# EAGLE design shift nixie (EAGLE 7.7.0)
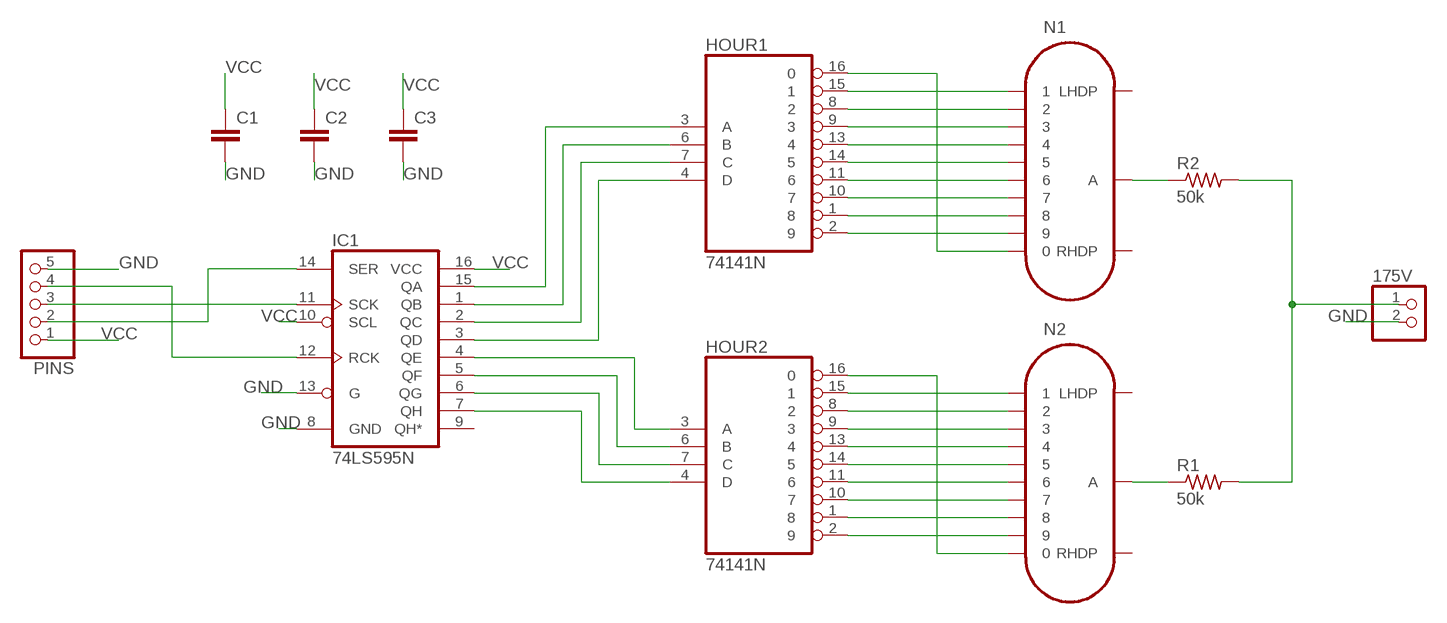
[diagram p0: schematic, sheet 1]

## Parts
175V  PINHD-1X2  [1X02]
C1  CAPPTH  [CAP-PTH-SMALL]
C2  CAPPTH  [CAP-PTH-SMALL]
C3  CAPPTH  [CAP-PTH-SMALL]
HOUR1  74141N  [DIL16]
HOUR2  74141N  [DIL16]
IC1  74LS595N  [DIL16]
N1  IN-14  [IN-14]
N2  IN-14  [IN-14]
PINS  PINHD-1X5  [1X05]
R1  50k  R-US_0204/7  [0204/7]
R2  50k  R-US_0204/7  [0204/7]

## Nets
GND: 175V.2 C1.2 C2.2 C3.2 IC1.8(GND) IC1.13(G) PINS.5
N$1: IC1.11(SCK) PINS.3
N$2: IC1.14(SER) PINS.2
N$3: IC1.12(RCK) PINS.4
N$4: HOUR1.3(A) IC1.15(QA)
N$5: HOUR1.6(B) IC1.1(QB)
N$6: HOUR1.7(C) IC1.2(QC)
N$7: HOUR1.4(D) IC1.3(QD)
N$8: HOUR2.3(A) IC1.4(QE)
N$9: HOUR2.6(B) IC1.5(QF)
N$10: HOUR2.7(C) IC1.6(QG)
N$11: HOUR2.4(D) IC1.7(QH)
N$12: HOUR2.15 N2.1
N$13: HOUR2.8 N2.2
N$14: HOUR2.9 N2.3
N$15: HOUR2.13 N2.4
N$16: HOUR2.14 N2.5
N$17: HOUR2.11 N2.6
N$18: HOUR2.10 N2.7
N$19: HOUR2.1 N2.8
N$20: HOUR2.2 N2.9
N$21: HOUR2.16 N2.0
N$22: HOUR1.15 N1.1
N$23: HOUR1.8 N1.2
N$24: HOUR1.9 N1.3
N$25: HOUR1.13 N1.4
N$26: HOUR1.14 N1.5
N$27: HOUR1.11 N1.6
N$28: HOUR1.10 N1.7
N$29: HOUR1.1 N1.8
N$30: HOUR1.2 N1.9
N$31: HOUR1.16 N1.0
N$32: N1.A R2.1
N$33: N2.A R1.1
N$35: 175V.1 R1.2 R2.2
VCC: C1.1 C2.1 C3.1 IC1.10(SCL) IC1.16(VCC) PINS.1
Unconnected: IC1.9(QH*) N1.LHDP N1.RHDP N2.LHDP N2.RHDP

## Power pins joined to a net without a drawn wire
GND: HOUR1.12(GND) HOUR2.12(GND)
VCC: HOUR1.5(VCC) HOUR2.5(VCC)

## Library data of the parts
175V = pinhead:PINHD-1X2: PIN HEADER
C1-C3 = SparkFun-Passives:CAP: Capacitor
HOUR1 HOUR2 = 74xx-eu:74*141: BCD to decimal DECODER/DRIVER
IC1 = SparkFun-DigitalIC:74*595: 8-bit SHIFT REGISTER, output latch
N1 N2 = russian-nixies:IN-14: IN-14: medium numeric frontview nixie tube
PINS = pinhead:PINHD-1X5: PIN HEADER
R1 R2 = resistor:R-US_: RESISTOR, American symbol

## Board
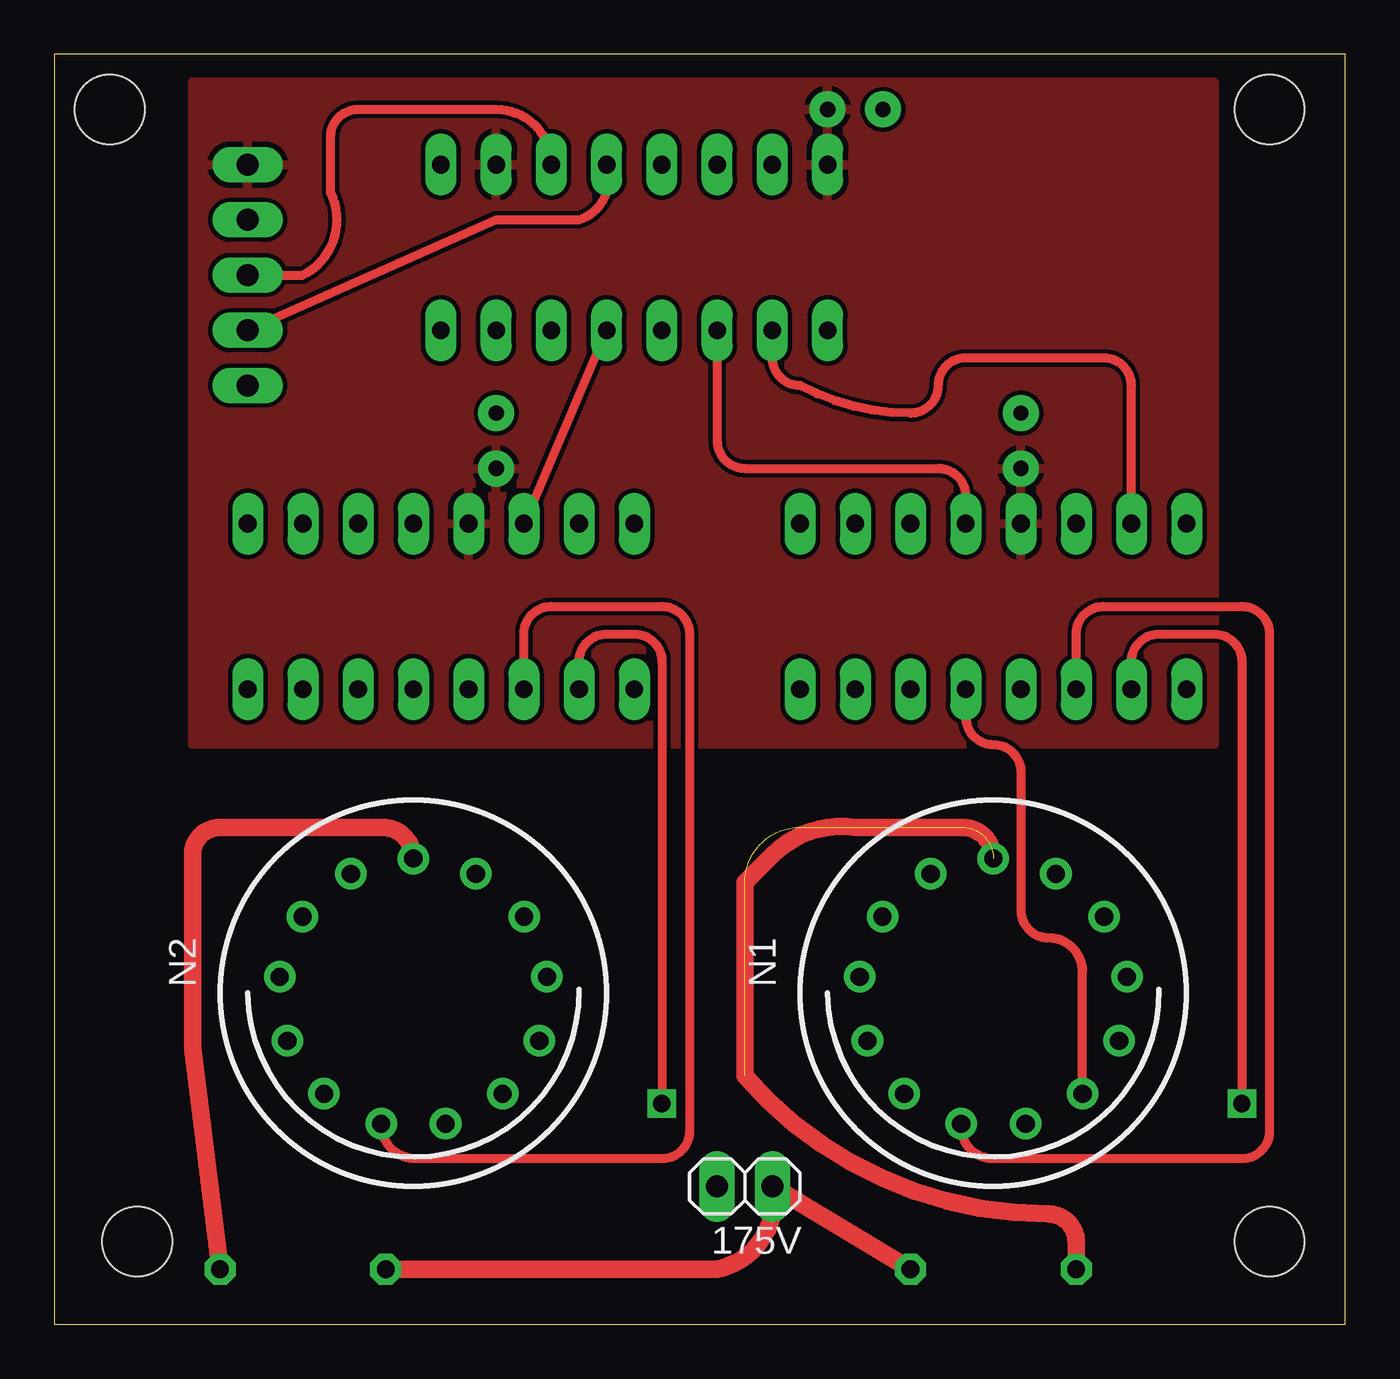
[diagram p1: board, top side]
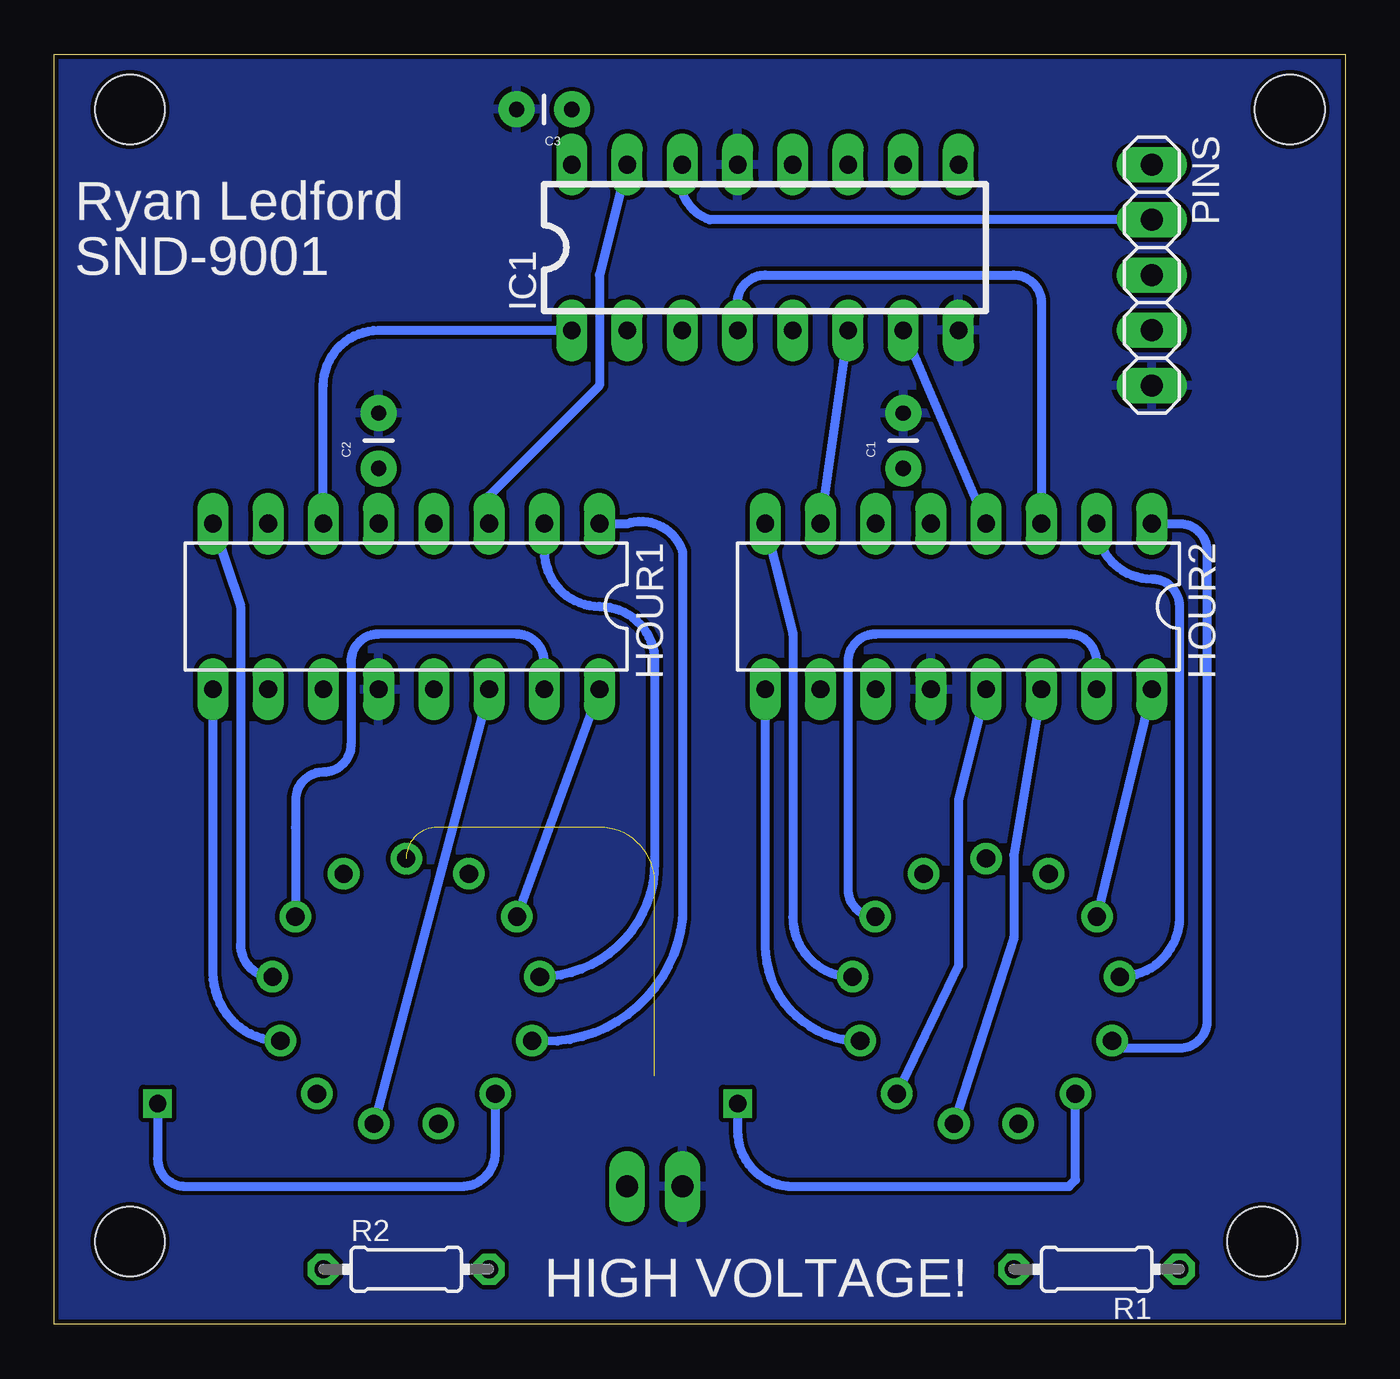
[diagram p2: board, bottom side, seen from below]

Size 59.36 x 58.41 mm. Coordinates in mm from the lower left corner, seen from the top.
Outline: 0,0 59.36,0 59.36,58.41 0,58.41 0,0
Copper layers (1*16): Top 0.035mm / dielectric 1.5mm / Bottom 0.035mm
Design rules "SparkFun": minimum track width 8mil, minimum drill 20mil, track to track 8mil, track to pad 8mil, pad to pad 8mil, via to via 8mil, smd to smd 8mil, copper to edge 8mil, drill to drill 8mil, minimum pad ring 12mil, minimum via ring 10mil, stop-mask expansion 4mil, vias tented up to drill 20mil, thermal gap 10mil
Holes 3.2 mm at 2.54,55.88 55.88,55.88 55.88,3.81 3.81,3.81

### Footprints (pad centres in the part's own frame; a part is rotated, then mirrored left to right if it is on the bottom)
1X02 = drill 1.016 long: 1 -1.27,0; 2 1.27,0
CAP-PTH-SMALL = drill 0.7 pad 1.651: 1 0,0; 2 2.54,0
DIL16 = drill 0.813 long: 1 -8.89,-3.81; 2 -6.35,-3.81; 3 -3.81,-3.81; 4 -1.27,-3.81; 5 1.27,-3.81; 6 3.81,-3.81; 7 6.35,-3.81; 8 8.89,-3.81; 9 8.89,3.81; 10 6.35,3.81; 11 3.81,3.81; 12 1.27,3.81; 13 -1.27,3.81; 14 -3.81,3.81; 15 -6.35,3.81; 16 -8.89,3.81
IN-14 = drill 0.84: 0 5.094,-3.516; 1 -5.094,-3.516; 2 -6.145,-0.746; 3 -5.788,2.195; 4 -4.105,4.633; 5 -1.481,6.01; 6 1.481,6.01; 7 4.105,4.633; 8 5.788,2.195; 9 6.145,-0.746; A 0,-6.19; LHDP 2.877,-5.481; RHDP -2.877,-5.481
1X05 = drill 1.016 long: 1 -5.08,0; 2 -2.54,0; 3 0,0; 4 2.54,0; 5 5.08,0
0204/7 = drill 0.813 octagon: 1 -3.81,0; 2 3.81,0

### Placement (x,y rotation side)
175V  31.75,6.35 180 top
C1  20.32,39.37 90 bottom
C2  44.45,39.37 90 bottom
C3  35.56,55.88 180 bottom
HOUR1  43.18,33.02 180 bottom
HOUR2  17.78,33.02 180 bottom
IC1  26.67,49.53 0 bottom
N1  43.18,15.24 180 top
N2  16.51,15.24 180 top
PINS  8.89,48.26 270 bottom
R1  11.43,2.54 180 bottom
R2  43.18,2.54 0 bottom

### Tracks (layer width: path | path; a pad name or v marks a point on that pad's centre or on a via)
GND
  pour Bottom: 53.34,57.15 53.34,26.67 6.35,26.67
  pour Bottom: -1.27,59.69 60.96,59.69 60.96,58.42 60.96,-1.27 -1.27,-1.27
N$1
  Top 0.406: PINS.3 11.43,48.26 arc90 12.7,52.07 12.7,54.61 arc-90 13.97,55.88 20.32,55.88 arc-90 IC1.11
N$2
  Bottom 0.406: PINS.2 29.21,50.8 arc90 IC1.14
N$3
  Top 0.406: PINS.4 20.32,50.8 24.13,50.8 arc90 IC1.12
N$4
  Bottom 0.406: IC1.15 34.29,48.26 34.29,43.18 39.37,38.1 HOUR1.3
N$5
  Bottom 0.406: HOUR1.6 46.99,43.18 arc90 44.45,45.72 IC1.1
N$6
  Top 0.406: HOUR1.7 49.53,43.18 arc90 48.26,44.45 41.91,44.45 arc90 40.64,43.18 arc-90 39.37,41.91 arc-28 34.29,43.18 arc-90 33.02,44.45 IC1.2
N$7
  Top 0.406: IC1.3 30.48,40.64 arc90 31.75,39.37 40.64,39.37 arc-90 41.91,38.1 HOUR1.4
N$8
  Bottom 0.406: IC1.4 27.94,46.99 arc90 26.67,48.26 15.24,48.26 arc90 13.97,46.99 HOUR2.3
N$9
  Top 0.406: IC1.5 HOUR2.6
N$10
  Bottom 0.406: IC1.6 HOUR2.7
N$11
  Bottom 0.406: IC1.7 HOUR2.4
N$12
  Bottom 0.406: HOUR2.15 11.43,30.48 arc-90 12.7,31.75 21.59,31.75 arc-90 22.86,30.48 22.86,20.01 arc-90 N2.1
N$13
  Bottom 0.406: HOUR2.8 25.4,31.75 25.4,18.73 arc-90 N2.2
N$14
  Bottom 0.406: HOUR2.9 26.67,17.42 arc-90 N2.3
N$15
  Bottom 0.406: HOUR2.13 17.78,24.13 17.78,16.51 N2.4
N$16
  Bottom 0.406: HOUR2.14 15.24,21.59 15.24,17.78 N2.5
N$17
  Top 0.406: HOUR2.11 21.59,31.75 arc-90 22.86,33.02 27.94,33.02 arc-90 29.21,31.75 29.21,8.89 arc-90 27.94,7.62 16.64,7.62 arc-90 N2.6
N$18  (via drill 0.8)
  Top 0.406: HOUR2.10 24.13,30.48 arc-90 25.4,31.75 26.67,31.75 arc-90 27.94,30.48 v27.94,10.16
  Bottom 0.406: v27.94,10.16 27.94,8.89 arc-90 25.4,6.35 12.7,6.35 12.41,6.65 N2.7
N$19
  Bottom 0.406: HOUR2.1 7.62,36.83 arc90 6.35,35.56 6.35,13.97 arc90 7.62,12.7 10.38,12.7 arc90 N2.8
N$20
  Bottom 0.406: HOUR2.2 arc-90 8.89,34.29 arc90 7.62,33.02 7.62,18.73 arc90 N2.9
N$21
  Bottom 0.406: HOUR2.16 N2.0
N$22
  Bottom 0.406: HOUR1.15 36.83,30.48 arc-90 38.1,31.75 44.45,31.75 arc-90 45.72,30.48 45.72,26.67 arc90 46.99,25.4 arc-90 48.26,24.13 48.26,22.86 arc-90 48.27,22.85 N1.1
N$23
  Bottom 0.406: HOUR1.8 50.8,33.02 50.8,17.46 arc-90 N1.2
N$24
  Bottom 0.406: HOUR1.9 52.07,16.15 arc-90 N1.3
N$25
  Top 0.406: N1.4 47.28,16.21 arc90 45.72,17.78 arc-90 44.45,19.05 44.45,25.4 arc90 43.18,26.67 arc-90 41.91,27.94 HOUR1.13
N$26
  Bottom 0.406: HOUR1.14 N1.5
N$27
  Top 0.406: HOUR1.11 46.99,31.75 arc-90 48.26,33.02 54.61,33.02 arc-90 55.88,31.75 55.88,8.89 arc-90 54.61,7.62 43.18,7.62 arc-90 41.7,9.1 N1.6
N$28  (via drill 0.8)
  Top 0.406: HOUR1.10 49.53,30.48 arc-90 50.8,31.75 53.34,31.75 arc-90 54.61,30.48 v54.61,10.16
  Bottom 0.406: v54.61,10.16 54.61,7.62 arc-90 53.34,6.35 40.64,6.35 arc-90 39.07,7.92 N1.7
N$29
  Bottom 0.406: HOUR1.1 33.02,36.83 arc90 30.48,35.56 30.48,18.69 arc90 N1.8
N$30
  Bottom 0.406: HOUR1.2 36.83,35.56 arc-90 34.29,33.02 arc90 31.75,30.48 31.75,21.27 arc90 N1.9
N$31
  Bottom 0.406: HOUR1.16 N1.0
N$32  (4 unrouted)
  Top 0.813: R2.1 46.99,3.81 arc90 45.72,5.08 arc-49 31.75,11.43 31.75,20.32 33.02,21.59 arc-53 36.83,22.86 41.75,22.86 arc-90 N1.A
N$33
  Top 0.813: R1.1 6.35,12.7 6.35,21.59 arc-90 7.62,22.86 15.08,22.86 arc-90 N2.A
N$35
  Top 0.813: R2.2 175V.1 arc-90 30.48,2.54 R1.2
VCC
  pour Top: 6.35,57.15 53.34,57.15 53.34,55.88 53.34,26.67 6.35,26.67

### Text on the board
bPlace: Ryan Ledford | SND-9001 | HIGH VOLTAGE!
